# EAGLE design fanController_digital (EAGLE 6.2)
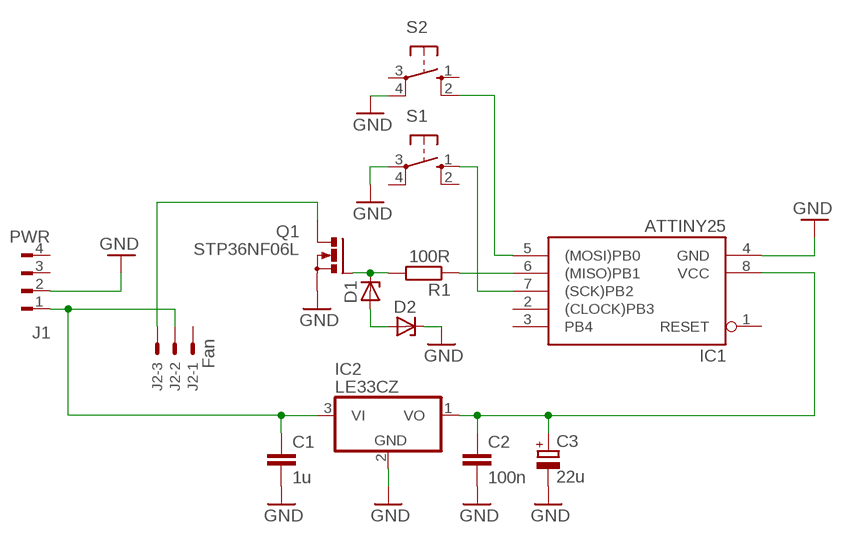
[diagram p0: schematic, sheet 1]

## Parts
C1  1u  C2.5/2  [C2.5-2]
C2  100n  C2.5/2  [C2.5-2]
C3  22u  CPOL-EUE2-4  [E2-4]
D1  ZENER-DIODEZD-5  [ZDIO-5]
D2  ZENER-DIODEZD-5  [ZDIO-5]
IC1  ATTINY25  TINY22P  [DIL08]
IC2  LE33CZ  78L05Z  [TO92]
J1  PWR  FLOP-4W827001  [827001]
J2  Fan  22-23-2031  [22-23-2031]
Q1  STP36NF06L  BUZ11BV  [TO220BV]
R1  100R  R-EU_0207/7  [0207/7]
S1  10-XX  [B3F-10XX]
S2  10-XX  [B3F-10XX]

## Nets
GND: C1.2 C2.2 C3.- D2.C IC1.4(GND) IC2.2(GND) J1.2 Q1.S S1.3(P) S2.4(P1)
N$1: D1.C Q1.G R1.2
N$2: C1.1 IC2.3(VI) J1.1 J2.2
N$3: IC1.5((MOSI)PB0) S2.2(S1)
N$5: IC1.7((SCK)PB2) S1.1(S)
N$6: IC1.6((MISO)PB1) R1.1
N$7: D1.A D2.A
N$9: J2.3 Q1.D
VCC: C2.1 C3.+ IC1.8(VCC) IC2.1(VO)
Unconnected: IC1.1(RESET) IC1.2((CLOCK)PB3) IC1.3(PB4) J1.3 J1.4 J2.1 S1.2(S1) S1.4(P1) S2.1(S) S2.3(P)

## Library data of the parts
C1 C2 = capacitor-wima:C: CAPACITOR
C3 = rcl:CPOL-EU: POLARIZED CAPACITOR, European symbol
D1 D2 = diode:ZENER-DIODE: Z-Diode
IC1 = atmel:TINY22: MICROCONTROLLER 1K ROM 128 bytes RAM 128 bytes EEPROM; OC_FARNELL: unknown; OC_NEWARK: unknown
IC2 = linear:78*: Positive VOLTAGE REGULATOR Source: http://cache.national.com/ds/LM/LM78L05.pdf http://www.fairchildsemi.com/ds/LM/LM7805.pdf
J1 = con-amp:FLOP-4W: MATE N-LOCK Floppy / HDD conector Distributor: Bürklin 71F972
J2 = con-molex:22-23-2031: .100" (2.54mm) Center Header - 3 Pin; MF: MOLEX; MPN: 22-23-2031; OC_FARNELL: 1462950; OC_NEWARK: 30C0862
Q1 = transistor-power:BUZ11: N-CHANNEL MOS FET
R1 = resistor:R-EU_: RESISTOR, European symbol
S1 S2 = switch-omron:10-XX: OMRON SWITCH; MPN: B3F-1000; OC_FARNELL: 176432; OC_NEWARK: 36M3542

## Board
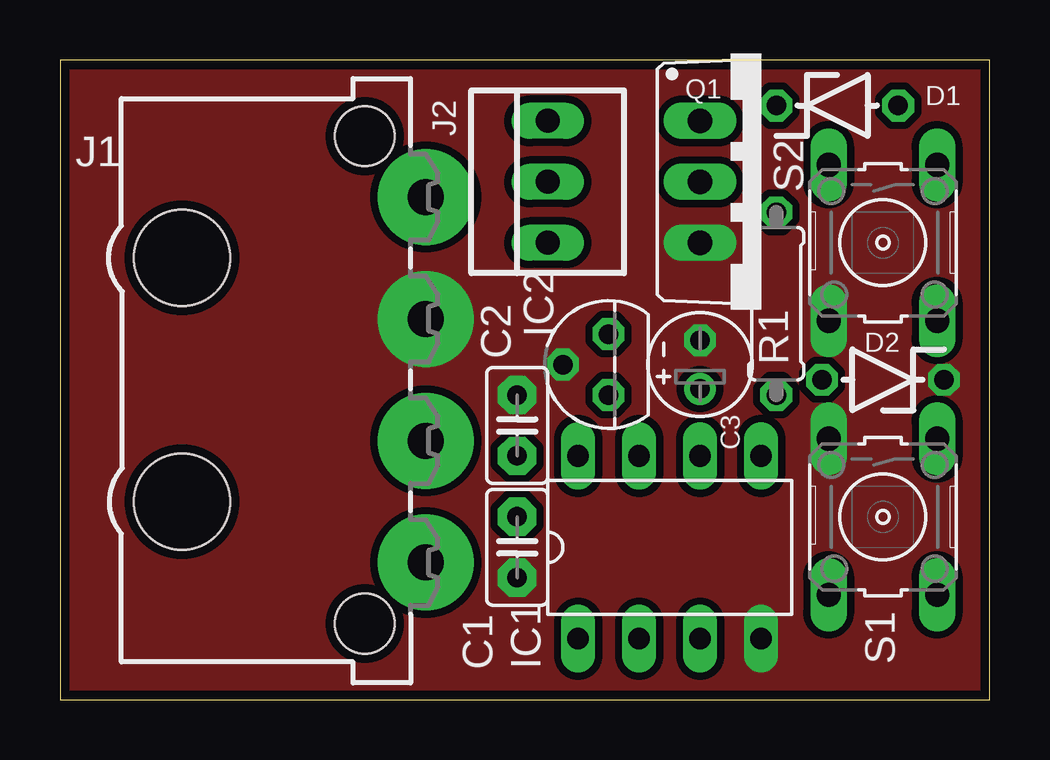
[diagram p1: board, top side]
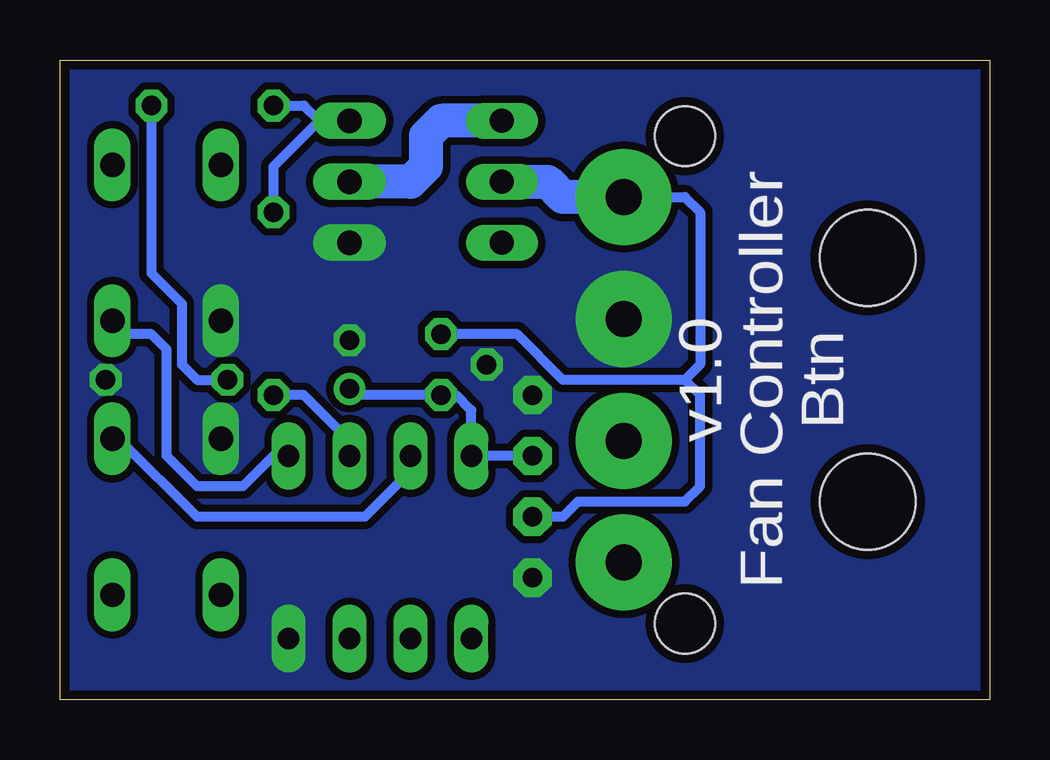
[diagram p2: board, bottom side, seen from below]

Size 38.73 x 26.67 mm. Coordinates in mm from the lower left corner, seen from the top.
Outline: 0,0 38.73,0 38.73,26.67 0,26.67 0,0
Copper layers (1*16): Top 0.0356mm / dielectric 1.5011mm / Bottom 0.0356mm
Design rules: minimum track width 6mil, minimum drill 13mil, track to track 6mil, track to pad 6mil, pad to pad 6mil, via to via 6mil, smd to smd 6mil, copper to edge 15mil, drill to drill 6mil, minimum pad ring 10mil, minimum via ring 7mil, stop-mask expansion 4mil, vias tented up to drill 0mil, thermal gap 10mil

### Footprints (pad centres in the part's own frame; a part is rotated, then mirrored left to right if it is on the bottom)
C2.5-2 = drill 0.813 pad 1.6 octagon: 1 -1.27,0; 2 1.27,0
E2-4 = drill 0.813 pad 1.27: + -1.016,0 | drill 0.813 pad 1.27 octagon: - 1.016,0
ZDIO-5 = drill 0.813 octagon: A 2.54,0; C -2.54,0
DIL08 = drill 0.9 long: 1 -3.81,-3.81; 2 -1.27,-3.81; 3 1.27,-3.81; 4 3.81,-3.81; 5 3.81,3.81; 6 1.27,3.81; 7 -1.27,3.81; 8 -3.81,3.81
TO92 = drill 0.813 octagon: 1 -1.27,0; 2 0,1.905; 3 1.27,0
827001 = drill 1.5 pad 4: 1 -7.62,0; 2 -2.54,0; 3 2.54,0; 4 7.62,0 | hole 4: 5.08,-10.16; -5.08,-10.16 | hole 2.5: 10.16,-2.54; -10.16,-2.54
22-23-2031 = drill 1 long: 1 -2.54,0; 2 0,0; 3 2.54,0
TO220BV = drill 1.016 long: D 0,-2.54; G -2.54,-2.54; S 2.54,-2.54
0207/7 = drill 0.813 octagon: 1 -3.81,0; 2 3.81,0
B3F-10XX = drill 1.016 long: 1 -3.251,2.261; 2 3.251,2.261; 3 -3.251,-2.261; 4 3.251,-2.261

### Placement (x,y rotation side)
C1  19.05,6.35 270 top
C2  19.05,11.43 90 top
C3  26.67,13.97 90 top
D1  32.38,24.77 0 top
D2  34.29,13.34 180 top
IC1  25.4,6.35 0 top
IC2  22.86,13.97 90 top
J1  15.24,13.34 270 top
J2  20.32,21.59 90 top
Q1  29.21,21.59 270 top
R1  29.84,16.51 90 top
S1  34.29,7.62 270 top
S2  34.29,19.05 270 top

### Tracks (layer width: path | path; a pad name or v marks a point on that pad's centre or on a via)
GND
  pour Bottom (isolate 0.305, no thermals): 0,26.67 38.73,26.67 38.73,0 0,0
  pour Top (isolate 0.305, no thermals): 0,26.67 38.73,26.67 38.73,0 0,0
N$1
  Bottom 0.406: 27.94,24.13 29.84,22.23 R1.2 | 27.94,24.13 Q1.G | D1.C 28.57,24.77 27.94,24.13
N$2
  Bottom 0.406: IC2.3 19.68,15.24 17.78,13.34 12.7,13.34 | 12.7,13.34 12.06,12.7 12.06,8.89 12.7,8.26 17.14,8.26 17.78,7.62 C1.1 | J1.1 12.7,20.95 12.06,20.32 12.06,13.97 12.7,13.34
  Bottom 1.422: J1.1 17.78,20.95 18.41,21.59 J2.2
N$3
  Bottom 0.406: S2.2 35.99,15.24 34.92,15.24 34.29,14.61 34.29,10.16 33.02,8.89 31.11,8.89 29.84,10.16 IC1.5
N$5
  Bottom 0.406: IC1.7 24.13,9.53 26.04,7.62 33.02,7.62 36.2,10.79 36.47,10.79 S1.1
N$6
  Bottom 0.406: IC1.6 26.67,10.79 28.57,12.7 R1.1
N$7
  Bottom 0.406: D1.A 34.92,17.78 33.66,16.51 33.66,13.97 33.02,13.34 D2.A
N$9
  Bottom 1.422: J2.3 22.86,24.13 23.5,23.5 23.5,22.23 24.13,21.59 Q1.D
VCC
  Bottom 0.406: C2.1 IC1.8 21.59,12.06 22.23,12.7 IC2.1 26.67,12.7 C3.+

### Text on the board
bNames: Btn | Fan Controller | v1.0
